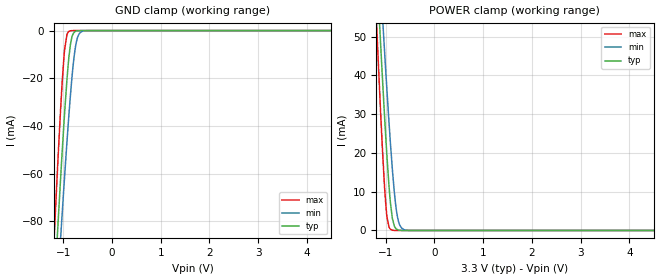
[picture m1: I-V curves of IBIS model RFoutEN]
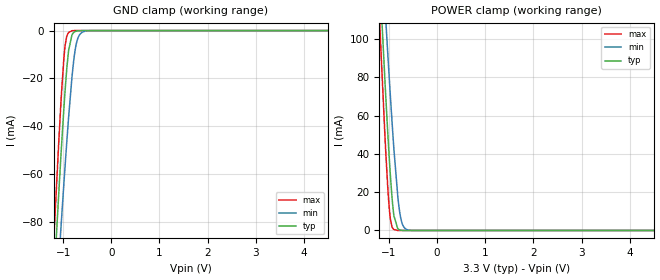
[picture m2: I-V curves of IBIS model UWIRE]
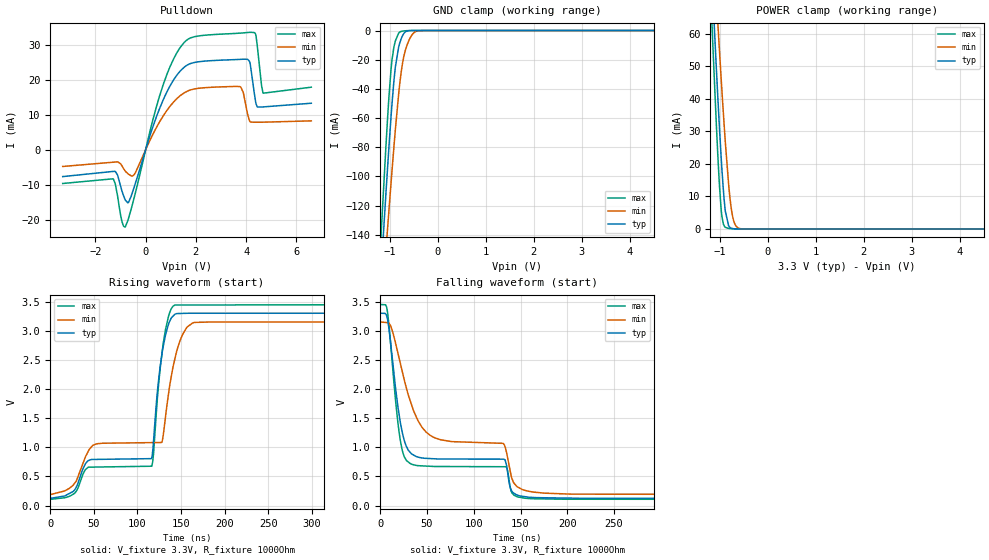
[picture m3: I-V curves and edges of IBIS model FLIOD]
| Texas Instruments Incorporated
| Low-Noise Clock Jitter Cleaner with Dual Loop PLLs
| Marketing part#   Voltage Range   Package-type   #pins/pkg drawing
| LMX2541SQ2060E   3.15V - 3.45V   WQFN   36-pin NJK
[IBIS Ver]   4.1
[File name]   lmx2541.ibs
[File Rev]   1.0
[Date]   04/19/2014
[Source]   Model built from spectre simulations at:
   Texas Instruments Incorporated.
   Analog-eLab, HPA
   12500 TI Blvd
   Dallas, TX -75243
   For Support e-mail: elab_ibis@list.ti.com
[Notes]   Revision History
   Rev 1.0: 04/19/2014
   - Pulldown non-monotonic on FLIOD, Open-drain output
   - Pulldown, Pullup non-monotonic on FLIOPP, Push-Pull output
   - No model provided for OSCIN. This is a crystal oscillator input, and requires special routing
   - No model provided for RFOUT. Open collector output with output impedence dependent on frequency.
   - Package level and pin level RLC not available
   - ccomp values are based on PVT settings:
   MIN: Low Voltage, High Temperature, Weak Process
   TYP: Nominal Voltage, Nominal Temperature, Nominal Process
   MAX: High Voltage, Low Temperature, Fast Process
   - C_comp although listed in numerical order of value are obtained from varying PVT conditions.
   For PVT conditions for each specific value, refer to the buffer description under respective [Model].
   IBIS model user is responsible for using appropriate C_comp to simulate for Signal Integrity.
[Disclaimer]  This model is designed as an aid for customers of Texas Instruments
 TI and its licensors and suppliers make no warranties, either expressed
 or implied, with respect to this  model, including the warranties of
 merchantability or fitness for a particular purpose.
 The model is provided solely on an "as is" basis. The entire risk as to
 its quality and performance is with the customer.
[Copyright] (C)Copyright 2014 Texas Instruments Incorporated.
   All rights reserved.
[Component]   LMX2541
[Manufacturer]  Texas Instruments Incorporated
[Package]   |36-pin WQFN NJK package
|   typ   min   max
R_pkg   0   0   0
L_pkg   0   0   0
C_pkg   0   0   0
[Pin]   signal_name   model_name   R_pin   L_pin   C_pin
1   GND   GND
2   VrefRFout   NC
3   VccRFout   NC
4   L1   NC
5   Lmid   NC
6   L2   NC
7   VccVCO   NC
8   VregVCO   NC
9   VrefVCO   NC
10   GND   GND
11   CE   UWIRE
12   ExtVCOin   NC
13   VccPLL1   NC
14   VccCP1   NC
15   Vtune   NC
16   CPout   NC
17   FLout   FLOUT
18   VccCP2   NC
19   VccPLL2   NC
20   Ftest/LD   FLIO
21   OSCIN   NC
22   OSCIN*   NC
23   VccOSCin   NC
24   RFoutEN   RFoutEN
25   VccFRAC   NC
26   VregFRAC   NC
27   GND   GND
28   VccDig   POWER
29   VccBias   POWER
30   Bypass   NC
31   VccDiv   NC
32   DATA   UWIRE
33   CLK   UWIRE
34   LE   UWIRE
35   NC   NC
36   RFOUT   NC
|   Model Selector statement
[Model Selector] FLIO
FLIOPP   Ftest/LD in push-pull configuration
FLIOD   Ftest/LD in open-drain configuration
| Models and submodels in the file (5): RFoutEN (Input), UWIRE (Input), FLIOD (Open_drain), FLIOPP (3-state), FLOUT (Output)
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|   Model RFoutEN
[Model]   RFoutEN
Model_type   Input
Vinl = 0.4
Vinh = 1.6
|   typ   min   max
|   (nom PVT)   (fast PVT)   (slow PVT)
C_comp   0.3093pF   0.3093pF   0.3093pF
[Voltage Range]   3.3   3.15   3.45
[Temperature Range]   27   125   -40
[Power Clamp Reference]   3.3   3.15   3.45
[GND Clamp Reference]   0   0   0
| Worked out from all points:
|   GND clamp passes 1 mA (typ) near -0.79 V on its own axis
|   POWER clamp passes 1 mA (typ) near -0.82 V on its own axis
[GND Clamp]
|   Voltage   I(typ)   I(min)   I(max)
-3.3V     -965.6mA   -893.6mA   -1.069A
-1.181V   -108.3mA   -129.3mA   -84.35mA
-1.112V   -82.59mA   -106mA     -55.39mA
-1.043V   -57.82mA   -83.32mA   -28.72mA
-973.5mV  -34.81mA   -61.42mA   -8.124mA
-924mV    -20.4mA    -46.56mA   -1.597mA
-884.4mV  -11.09mA   -35.36mA   -347uA
-825mV    -2.889mA   -20.4mA    -26.1uA
-745.8mV  -310.8uA   -6.404mA   -528.4nA
-676.5mV  -33.31uA   -1.499mA   -14.52nA
-577.5mV  -943.1nA   -148.2uA   0A
6.59V     0A         0A         0A
[POWER Clamp]
|   Voltage   I(typ)   I(min)   I(max)
-3.3V     638.8mA    590.5mA    708.3mA
-1.191V   69.15mA    82.63mA    53.96mA
-1.181V   66.68mA    80.4mA     51.15mA
-1.102V   47.28mA    62.82mA    29.5mA
-1.033V   31.21mA    47.91mA    12.87mA
-993.3mV  22.67mA    39.68mA    5.73mA
-933.9mV  11.5mA     27.94mA    888.7uA
-864.6mV  3.112mA    15.73mA    67.37uA
-805.2mV  711.5uA    7.563mA    4.089uA
-745.8mV  145.3uA    2.701mA    212.4nA
-577.5mV  412.5nA    72uA       0A
6.59V     0A         0A         0A
|   Model UWIRE
[Model]   UWIRE
Model_type   Input
Vinl = .8
Vinh = 2
|   typ   min   max
|   (nom PVT)   (fast PVT)   (slow PVT)
C_comp   0.307p   0.300pF   0.311pF
| Where   nom PVT is  Nominal Process, 3.3V, 27C
|   Fast PVT is Strong Process, 3.45V, -40C
|   Slow PVT is Weak Process, 3.15V, 125C
[Voltage Range]   3.3   3.15   3.45
[Temperature Range]   27   125   -40
[Power Clamp Reference]   3.3   3.15   3.45
[GND Clamp Reference]   0   0   0
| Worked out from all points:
|   GND clamp passes 1 mA (typ) near -0.79 V on its own axis
|   POWER clamp passes 1 mA (typ) near -0.82 V on its own axis
[GND Clamp]
|   Voltage   I(typ)   I(min)   I(max)
-3.3V     -942.6mA   -854.7mA   -1.024A
-1.184V   -101.6mA   -126.3mA   -83.34mA
-1.085V   -65.79mA   -94.69mA   -44.16mA
-1.045V   -52.12mA   -82.34mA   -29.83mA
-976mV    -29.87mA   -61.37mA   -9.537mA
-926.5mV  -16.4mA    -47.1mA    -2.511mA
-886.9mV  -8.33mA    -36.31mA   -808.9uA
-817.6mV  -1.836mA   -19.65mA   -81.57uA
-758.2mV  -487.9uA   -9.126mA   -5.867uA
-698.8mV  -104.9uA   -3.449mA   -310.4nA
-510.7mV  -111.1nA   -127.1uA   0A
6.598V    0A         0A         0A
[POWER Clamp]
|   Voltage   I(typ)   I(min)   I(max)
-3.3V     1.303A     1.181A     1.417A
-1.194V   133.3mA    166.4mA    109.3mA
-1.174V   123.1mA    157.5mA    98.12mA
-1.085V   78.84mA    118.1mA    50.11mA
-1.065V   69.42mA    109.5mA    40.33mA
-985.9mV  34.63mA    76.33mA    9.435mA
-896.8mV  7.626mA    42.28mA    483.8uA
-817.6mV  959.4uA    18.05mA    15.01uA
-768.1mV  226.4uA    8.204mA    1.297uA
-708.7mV  27.84uA    2.579mA    63.14nA
-599.8mV  421.7nA    251.8uA    0A
6.598V    0A         0A         0A
|   Model FLIOD
[Model]   FLIOD
Model_type   Open_drain
Polarity   Non-Inverting
Vmeas = 1.65
Vref = 3.3
Cref = 15pF
Rref = 1000
|   typ   min   max
|   (nom PVT)   (fast PVT)   (slow PVT)
C_comp   0.430p   0.415p   0.443p
|C_comp (ON state)   0.430p   0.415p   0.443p
|C_comp (OFF state)   0.432p   0.420p   0.446p
[Voltage Range]   3.3   3.15   3.45
[Temperature Range]   27   125   -40
[Pullup Reference]   3.3   3.15   3.45
[Pulldown Reference]   0   0   0
[Power Clamp Reference]   3.3   3.15   3.45
[GND Clamp Reference]   0   0   0
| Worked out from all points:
|   slope of the pulldown table from 0 to 0.495 V, typ, clamps not added: 46.3 ohm
|   GND clamp passes 1 mA (typ) near -0.68 V on its own axis
|   POWER clamp passes 1 mA (typ) near -0.82 V on its own axis
|   falling waveform, V_fixture 3.3V, R_fixture 1000Ohm: 20-80 % time 122ns typ, 117ns min, 16.8ns max; typ from 3.3 V to 0.124 V
|   rising waveform, V_fixture 3.3V, R_fixture 1000Ohm: 20-80 % time 86.2ns typ, 105ns min, 11.9ns max; typ from 0.124 V to 3.3 V
[Pulldown]
|   Voltage   I(typ)   I(min)   I(max)
-3.3V     -7.679mA   -4.774mA   -9.657mA
-1.293V   -6.194mA   -3.552mA   -8.311mA
-807.7mV  -14.42mA   -6.13mA    -22.12mA
-451.3mV  -10.61mA   -7.078mA   -13.61mA
736.7mV   14.92mA    10.13mA    19.44mA
1.816V    24.84mA    17.26mA    32.19mA
3.776V    25.97mA    18.09mA    33.5mA
4.063V    25.97mA    10.18mA    33.68mA
4.33V     16.1mA     7.922mA    33.67mA
4.449V    12.29mA    7.926mA    29.63mA
4.677V    12.32mA    7.938mA    16.26mA
6.598V    13.37mA    8.316mA    17.98mA
[GND Clamp]
|   Voltage   I(typ)   I(min)   I(max)
-3.3V     -1.383A    -1.212A    -1.541A
-1.184V   -165.8mA   -196.6mA   -140.6mA
-1.164V   -155.1mA   -187.6mA   -128.4mA
-1.085V   -113.1mA   -152mA     -80.86mA
-1.045V   -92.77mA   -134.5mA   -58.76mA
-966.1mV  -54.82mA   -100.5mA   -23.33mA
-886.9mV  -25.31mA   -68.43mA   -7.255mA
-778mV    -6.955mA   -32.12mA   -785uA
-718.6mV  -2.526mA   -19.33mA   -330.1uA
-639.4mV  -313.3uA   -9.741mA   -94.29uA
-401.8mV  -461.1nA   -145.3uA   -134.8nA
6.598V    0A         0A         0A
[POWER Clamp]
|   Voltage   I(typ)   I(min)   I(max)
-3.3V     787.6mA    691.1mA    878.1mA
-1.164V   76.78mA    94.56mA    62.67mA
-1.154V   73.73mA    91.97mA    59.2mA
-1.075V   49.88mA    71.51mA    32.58mA
-1.035V   38.51mA    61.52mA    20.57mA
-966.1mV  20.36mA    44.61mA    4.96mA
-886.9mV  5.513mA    26.79mA    507.5uA
-807.7mV  734uA      12.17mA    150.8uA
-748.3mV  159.3uA    4.962mA    78.71uA
-688.9mV  45.34uA    1.579mA    33.67uA
-589.9mV  6.415uA    160.7uA    3.88uA
6.598V    0A         0A         0A
[Ramp]
R_load = 1000
|   typ   min   max
dV/dt_r   1.90551/8.61785e-08   1.77705/1.04499e-07   2.00559/1.1897e-08
dV/dt_f   1.9054/1.21981e-07   1.77705/1.16927e-07   2.00557/1.67816e-08
[Falling Waveform]
V_fixture = 3.3V
V_fixture_min = 3.15V
V_fixture_max = 3.45V
R_fixture = 1000Ohm
C_fixture = 0F
|   Time   V(typ)   V(min)   V(max)
0s        3.3V       3.15V      3.45V
6.834ns   3.254V     3.14V      3.405V
21.31ns   1.445V     2.451V     1.134V
32.38ns   906.2mV    1.781V     718.2mV
59.09ns   801.9mV    1.157V     670.9mV
131.9ns   796.5mV    1.06V      666.7mV
135.7ns   621.9mV    857.3mV    633.5mV
140.2ns   257.9mV    498.7mV    239.1mV
156.9ns   148.2mV    251.3mV    123.6mV
499.9ns   124.3mV    188.2mV    107.4mV
[Rising Waveform]
V_fixture = 3.3V
V_fixture_min = 3.15V
V_fixture_max = 3.45V
R_fixture = 1000Ohm
C_fixture = 0F
|   Time   V(typ)   V(min)   V(max)
0s        124.1mV    188.3mV    107.3mV
26.19ns   243mV      348.8mV    194.3mV
48.64ns   791.4mV    1.032V     660.4mV
116.4ns   817.1mV    1.08V      675.4mV
123.6ns   2.056V     1.082V     1.961V
129.5ns   2.724V     1.201V     2.774V
143ns     3.282V     2.519V     3.441V
151.9ns   3.297V     2.939V     3.441V
165.8ns   3.3V       3.143V     3.441V
499.9ns   3.3V       3.15V      3.45V
